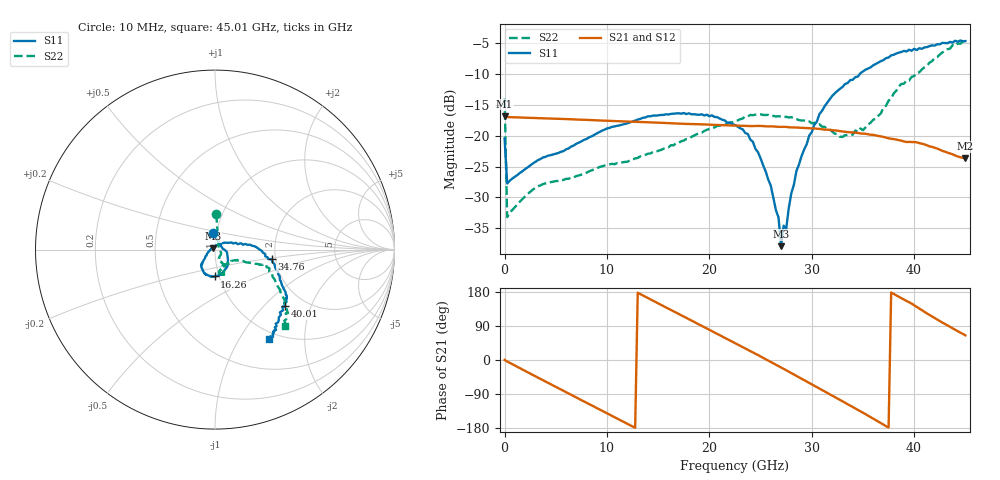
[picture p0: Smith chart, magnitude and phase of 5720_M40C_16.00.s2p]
! Device:  ADRF5720
! Description: 0.5dB LSB GaAs MMIC 6-bit Digital Attenuator
! Frequency:  0.000009 -  40 GHz
! Ports:
!	RF1	= Port 1
!	RF2	= Port 2
! Vdd:  3.3 Volt
! Vss:  -3.3 Volt
! Control:  0/3.3 Volt
! State:  16.00 dB attenuation
! Data:  The device was measured using G-S-G Probes on a matrix board.
!  Data was collected using an calibrated 4 port network analyzer.
!  The reference plane for this measurement is at the launchers.
! Note:  Analog Devices supplies this data as a sample of measured data
!  for this product.  Your particular data for this product may vary.
!  Data was taken at -40 degrees C.
!  Analog Devices reserves the right to change this data at anytime.
# GHZ S DB R 45.0
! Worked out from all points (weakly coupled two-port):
!   181 points, 10 MHz to 45.01 GHz, reference 45 ohm
!   highest |S21| = -16.83 dB at 10 MHz (marker M1); lowest = -23.7 dB at 45.01 GHz (marker M2)
!   lowest |S11| = -37.9 dB at 27.01 GHz (marker M3), VSWR 1.03, Z = 44.1 + j0.637 ohm
!   |S11| at or under -10 dB: start of sweep to 34.72 GHz
!   |S22| runs from -33.2 to -4.8 dB; largest |S21 - S12| = 0.00051
!   S11 on the Smith chart (normalised r, x): 10 MHz: 0.96, +0.18; 16.26 GHz: 0.95, -0.29; 34.76 GHz: 1.90, -0.23; 40.01 GHz: 1.59, -1.34; 45.01 GHz: 0.90, -1.35
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0.01  -20.50 98.4  -16.83 0.1  -16.85 0.1  -14.02 87.9
0.26  -27.75 12.8  -17.01 -3.9  -17.03 -3.9  -33.19 21.2
3.26  -23.97 -8.7  -17.18 -46.4  -17.20 -46.5  -28.19 -29.2
7.76  -20.69 -38.5  -17.45 -109.3  -17.47 -109.4  -26.13 -61.5
15.26  -16.66 -84.6  -17.93 145.9  -17.95 145.9  -22.34 -63.5
16.26  -16.49 -90.7  -18.02 131.9  -18.04 131.9  -21.55 -62.3
20.26  -16.73 -114.0  -18.25 76.1  -18.27 76.0  -18.78 -61.3
22.76  -18.55 -131.1  -18.39 41.0  -18.42 41.0  -17.55 -67.9
24.26  -21.01 -136.3  -18.46 20.1  -18.48 20.0  -16.70 -70.3
25.51  -25.82 -152.0  -18.50 1.8  -18.52 1.7  -16.67 -72.7
26.76  -33.23 161.7  -18.59 -16.1  -18.61 -16.3  -16.86 -75.4
27.01  -37.88 145.5  -18.59 -19.6  -18.61 -19.8  -16.92 -77.5
27.26  -34.57 120.7  -18.59 -23.3  -18.61 -23.5  -17.06 -76.6
27.51  -35.07 75.5  -18.59 -27.0  -18.61 -27.2  -16.95 -78.0
28.01  -29.33 50.6  -18.67 -34.2  -18.69 -34.4  -17.01 -79.2
28.51  -25.72 42.7  -18.70 -41.6  -18.73 -41.8  -17.33 -79.8
30.26  -18.23 18.1  -18.85 -67.7  -18.88 -67.8  -17.93 -78.9
32.76  -12.44 1.9  -19.28 -105.3  -19.30 -105.4  -20.19 -64.4
34.76  -9.91 -9.8  -19.65 -135.3  -19.67 -135.4  -18.84 -40.1
37.76  -7.03 -29.9  -20.52 178.1  -20.54 178.0  -13.99 -21.2
40.01  -5.97 -38.9  -21.05 144.5  -21.07 144.4  -10.36 -18.8
45.01  -4.72 -58.9  -23.69 65.0  -23.72 65.0  -4.77 -47.2
